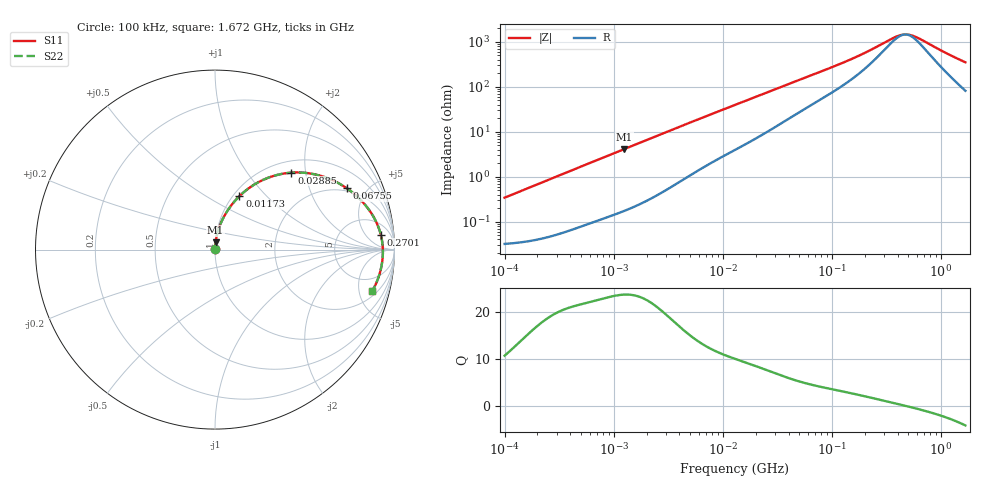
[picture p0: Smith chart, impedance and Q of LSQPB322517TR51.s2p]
! LSQPB322517TR51  S-PARAMETER MODEL  ( General Type )
! Model Generated by TAIYO YUDEN Corporation (http://www.ty-top.com)
! Version 1.0
! TAIYO YUDEN Control No. 100901NG22SB-FKC
! Copyright(c) 2010 TAIYO YUDEN CO.,LTD. All Rights Reserved.
! Product Description (link to TY-COMPAS)
! https://ds.yuden.co.jp/TYCOMPAS/or/detail?pn=LSQPB322517TR51M&u=M
! Products Name : Inductors
! Characteristics :
!  Inductance : 0.51 uH , SRF(min) : 270 MHz , DC Resistance(max) : 0.0377 Ohm
!  Rated Current : Saturation :3600 mA , Temp Rise : 2550 mA (40 degC)
!  Case Size : 3.2 x 2.5 / 0.126 x 0.098 [mm/inch] , Thickness : 1.7 / 0.068 [mm/inch]
!  (Conditions: Temperature = 25 degC , DC Bias Current/Voltage = 0A / 0V)
! External Node Assignments :
!  1  o---GGG---o  2
! GND o---------o GND
! Frequency Range : 0.1MHz  -  1672.468556MHz  [ 402 STEP ]
# MHz S RI R 50
! Freq[MHz].  S11 Real  S11 Imag  S21 Real  S21 Imag  S12 Real  S12 Imag  S22 Real  S22 Imag
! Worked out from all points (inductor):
!   401 points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, 100 kHz to 1.672 GHz, reference 50 ohm
!   read as one part in series: L = 539 nH near 105 kHz
!   highest Q = 23.6 at 1.253 MHz (marker M1), where L = 520 nH
!   self-resonance near 468.8 MHz
!   S11 on the Smith chart (normalised r, x): 100 kHz: 1.00, +0.01; 11.73 MHz: 1.07, +0.71; 28.85 MHz: 1.24, +1.67; 67.55 MHz: 1.83, +3.64; 270.1 MHz: 11, +13; 1.672 GHz: 2.62, -6.76
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0.1  0.00033 0.00339  0.9997 -0.00339  0.9997 -0.00339  0.00033 0.00339
0.509815  0.00107 0.0169  0.9989 -0.0169  0.9989 -0.0169  0.00107 0.0169
1.253352  0.00339 0.0407  0.9966 -0.0407  0.9966 -0.0407  0.00339 0.0407
2.599112  0.0109 0.0826  0.9891 -0.0826  0.9891 -0.0826  0.0109 0.0826
6.236302  0.0499 0.1835  0.9501 -0.1835  0.9501 -0.1835  0.0499 0.1835
11.73398  0.1361 0.2978  0.8639 -0.2978  0.8639 -0.2978  0.1361 0.2978
12.9324  0.1571 0.3171  0.8429 -0.3171  0.8429 -0.3171  0.1571 0.3171
18.62323  0.2594 0.3845  0.7406 -0.3845  0.7406 -0.3845  0.2594 0.3845
28.84736  0.4255 0.4287  0.5745 -0.4287  0.5745 -0.4287  0.4255 0.4287
41.54148  0.5729 0.4154  0.4271 -0.4154  0.4271 -0.4154  0.5729 0.4154
65.93127  0.7268 0.3469  0.2732 -0.3469  0.2732 -0.3469  0.7268 0.3469
67.55381  0.7335 0.3424  0.2665 -0.3424  0.2665 -0.3424  0.7335 0.3424
97.28049  0.817 0.2712  0.183 -0.2712  0.183 -0.2712  0.817 0.2712
143.5357  0.8761 0.1947  0.1239 -0.1947  0.1239 -0.1947  0.8761 0.1947
270.0712  0.9237 0.0837  0.0763 -0.0837  0.0763 -0.0837  0.9237 0.0837
336.1274  0.9307 0.0496  0.0693 -0.0496  0.0693 -0.0496  0.9307 0.0496
388.9146  0.9335 0.0277  0.0665 -0.0277  0.0665 -0.0277  0.9335 0.0277
439.1837  0.9349 0.00966  0.0651 -0.00966  0.0651 -0.00966  0.9349 0.00966
533.4742  0.9354 -0.0192  0.0646 0.0192  0.0646 0.0192  0.9354 -0.0192
632.4441  0.9341 -0.0451  0.0659 0.0451  0.0659 0.0451  0.9341 -0.0451
1189.982  0.9105 -0.1556  0.0895 0.1556  0.0895 0.1556  0.9105 -0.1556
1672.469  0.877 -0.2299  0.123 0.2299  0.123 0.2299  0.877 -0.2299
